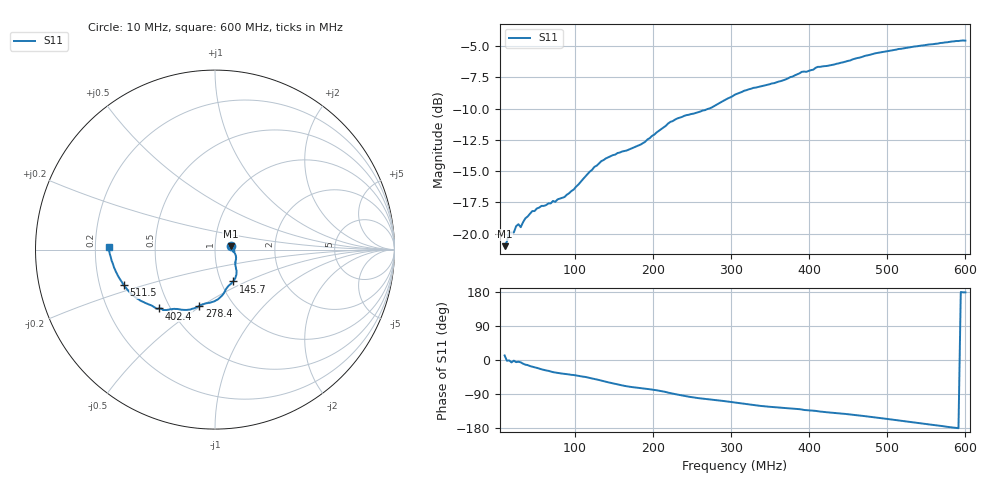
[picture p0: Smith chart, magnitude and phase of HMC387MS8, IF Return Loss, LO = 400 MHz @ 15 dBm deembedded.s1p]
!Hittite Microwave Corporation
!12 Elizabeth Drive
!Chelmsford, MA 01824
!Tel: 978-250-3343
!Fax: 978-250-3373
!Device: HMC387MS8, 450-500 MHz, GaAs MMIC High IP3 Mixer in 8-lead plastic SMT package
!Misc: IF Return Loss, LO = 400 MHz @ 15 dBm, Room
# MHZ S MA R 50
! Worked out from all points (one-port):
!   201 points, 10 MHz to 600 MHz, reference 50 ohm
!   lowest |S11| = -21.0 dB at 10 MHz (marker M1), VSWR 1.20, Z = 59.5 + j2.22 ohm
!   |S11| at or under -10 dB: start of sweep to 271.4 MHz
!   S11 on the Smith chart (normalised r, x): 10 MHz: 1.19, +0.04; 145.7 MHz: 1.14, -0.42; 278.4 MHz: 0.70, -0.49; 402.4 MHz: 0.44, -0.36; 511.5 MHz: 0.30, -0.17; 600 MHz: 0.26, +0.01
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10  0.089 12.0
12.95  0.093 -1.9
15.9  0.101 -1.1
18.85  0.101 -6.4
21.8  0.101 -1.7
27.7  0.109 -4.5
30.65  0.106 -6.3
36.55  0.115 -12.3
45.4  0.123 -17.7
83.75  0.139 -35.9
98.5  0.15 -39.6
125.05  0.185 -50.0
145.7  0.204 -60.3
157.5  0.211 -65.7
184.05  0.227 -74.0
207.65  0.258 -80.9
231.25  0.289 -91.2
278.45  0.324 -105.5
305  0.36 -112.1
337.45  0.388 -121.1
378.75  0.425 -128.0
402.35  0.451 -133.4
452.5  0.493 -143.6
482  0.524 -150.8
511.5  0.545 -158.6
526.25  0.555 -162.9
567.55  0.579 -173.7
600  0.592 178.5
